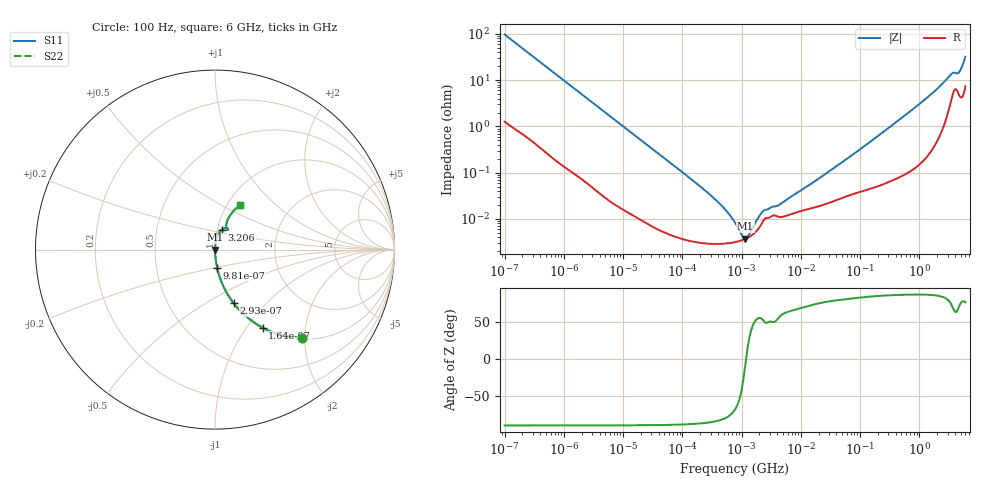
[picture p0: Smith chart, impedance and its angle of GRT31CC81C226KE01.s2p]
!Murata Part Number: GRT31CC81C226KE01
!These Parameters are Measured in Series Mode Connection
!Data Generated on Jun 19, 2026
!  o--ll--o
!Port1  Port2
!  o------o
!Operation Temp=25[degC], DC Bias Voltage=0[V]
!Freq. Start=100[Hz] Stop=6[GHz] 401[Steps]
# Hz S RI R 50
!Freq.(Hz) S11(Real) S11(Imag) S21(Real) S21(Imag) S12(Real) S12(Imag) S22(Real) S22(Imag)
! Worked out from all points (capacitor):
!   401 points, 100 Hz to 6 GHz, reference 50 ohm
!   read as one part in series: C = 16.3 uF near 109 Hz
!   lowest |Z| = 3.74 mohm at 1.159 MHz (marker M1)
!   series resonance near 1.19 MHz, so ESL is about 1.1 nH
!   S11 on the Smith chart (normalised r, x): 100 Hz: 1.03, -1.95; 164 Hz: 1.02, -1.19; 293 Hz: 1.01, -0.67; 981 Hz: 1.00, -0.20; 3.206 GHz: 1.05, +0.24; 6 GHz: 1.15, +0.62
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100  0.4868 -0.4934  0.5132 0.4934  0.5132 0.4934  0.4868 -0.4934
164  0.2657 -0.435  0.7343 0.435  0.7343 0.435  0.2657 -0.435
293  0.1046 -0.299  0.8954 0.299  0.8954 0.299  0.1046 -0.299
479  0.0432 -0.1966  0.9568 0.1966  0.9568 0.1966  0.0432 -0.1966
981  0.0115 -0.0999  0.9885 0.0999  0.9885 0.0999  0.0115 -0.0999
2008  0.00319 -0.0496  0.9968 0.0496  0.9968 0.0496  0.00319 -0.0496
40335  6.39e-05 -0.00254  0.9999 0.00254  0.9999 0.00254  6.39e-05 -0.00254
264476  2.94e-05 -0.000373  1 0.000373  1 0.000373  2.94e-05 -0.000373
452617  2.9e-05 -0.000196  1 0.000196  1 0.000196  2.9e-05 -0.000196
677235  3.05e-05 -0.000104  1 0.000104  1 0.000104  3.05e-05 -0.000104
774597  3.15e-05 -7.73e-05  1 7.73e-05  1 7.73e-05  3.15e-05 -7.73e-05
1159002  3.71e-05 -4.6e-06  1 4.6e-06  1 4.6e-06  3.71e-05 -4.6e-06
1813585  5.56e-05 7.69e-05  0.9999 -7.69e-05  0.9999 -7.69e-05  5.56e-05 7.69e-05
2372521  9.47e-05 0.000119  0.9999 -0.000119  0.9999 -0.000119  9.47e-05 0.000119
4246196  0.000111 0.000165  0.9999 -0.000165  0.9999 -0.000165  0.000111 0.000165
1.555665e7  0.000172 0.00057  0.9998 -0.00057  0.9998 -0.00057  0.000172 0.00057
3.124326e8  0.000726 0.00953  0.9993 -0.00953  0.9993 -0.00953  0.000726 0.00953
1.431855e9  0.00439 0.0442  0.9956 -0.0442  0.9956 -0.0442  0.00439 0.0442
3.205649e9  0.0373 0.1115  0.9627 -0.1115  0.9627 -0.1115  0.0373 0.1115
3.666503e9  0.062 0.12  0.938 -0.12  0.938 -0.12  0.062 0.12
4.586474e9  0.0639 0.12  0.9361 -0.12  0.9361 -0.12  0.0639 0.12
6e9  0.1411 0.2494  0.8589 -0.2494  0.8589 -0.2494  0.1411 0.2494
